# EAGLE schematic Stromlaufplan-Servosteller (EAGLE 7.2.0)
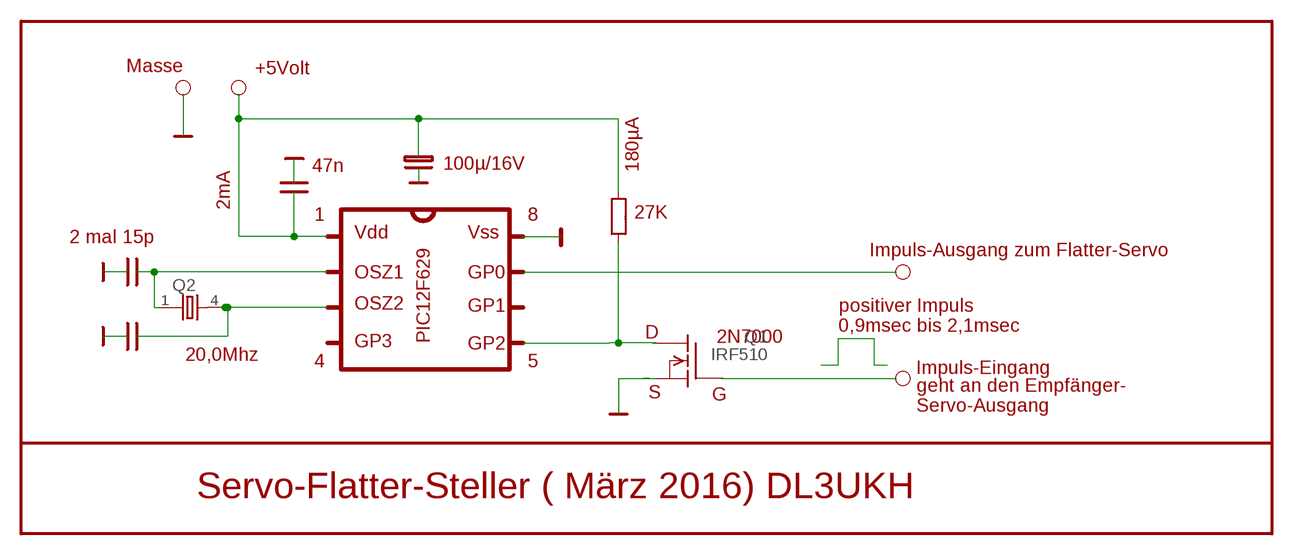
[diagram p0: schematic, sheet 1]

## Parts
Q1  IRF510  [TO220]
Q2  86SMX  [86SMX]

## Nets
N$6: Q1.2(D)
N$8: Q1.3(S)
N$9: Q1.1(G)
N$11: Q2.4
N$12: Q2.1

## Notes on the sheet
- Masse | +5Volt
- 47n | 100µ/16V | 180µA
- 2mA
- 1 | 8 | 27K
- 2 mal 15p
- Vdd | Vss
- Impuls-Ausgang zum Flatter-Servo
- OSZ1 | GP0
- OSZ2 | GP1 | positiver Impuls
- 0,9msec bis 2,1msec
- PIC12F629 | D | 2N7000
- 20,0Mhz | GP3 | GP2
- 4 | 5
- Impuls-Eingang
- geht an den Empfänger-
- S | G
- Servo-Ausgang
- Servo-Flatter-Steller ( März 2016) DL3UKH

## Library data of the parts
Q1 = transistor-fet:IRF510: N-Channel Enhancement MOSFET (HEXFET); 100V; 5,6A; 0,54Ohm
Q2 = crystal:86SMX: CRYSTAL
